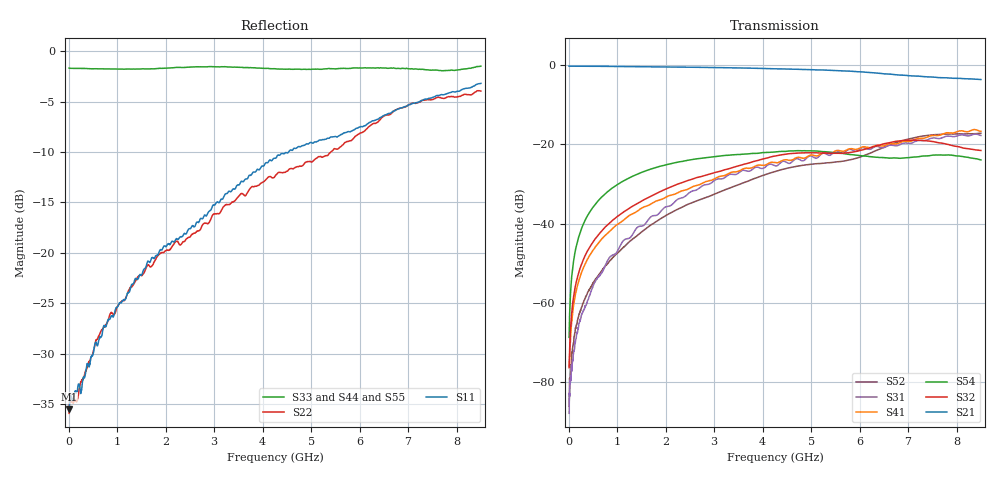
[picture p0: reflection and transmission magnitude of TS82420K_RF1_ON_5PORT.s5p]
!Created with skrf (http://scikit-rf.org).
# GHz S RI R 50.0
!freq ReS11 ImS11 ReS12 ImS12 ReS13 ImS13
! ReS14 ImS14 ReS15 ImS15
! ReS21 ImS21 ReS22 ImS22 ReS23 ImS23
! ReS24 ImS24 ReS25 ImS25
! ReS31 ImS31 ReS32 ImS32 ReS33 ImS33
! ReS34 ImS34 ReS35 ImS35
! ReS41 ImS41 ReS42 ImS42 ReS43 ImS43
! ReS44 ImS44 ReS45 ImS45
! ReS51 ImS51 ReS52 ImS52 ReS53 ImS53
! ReS54 ImS54 ReS55 ImS55
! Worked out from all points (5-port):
!   1601 points, 10 MHz to 8.5 GHz, reference 50 ohm
!   strongest paths, dB at 10 MHz, 2.132 GHz, 4.255 GHz, 6.378 GHz, 8.5 GHz:
!     S21: -0.2, -0.4, -0.9, -2.0, -3.6
!     S32: -76.4, -30.6, -22.9, -20.2, -21.5
!     S54: -68.8, -24.8, -21.9, -23.2, -23.9
!     S41: -76.0, -32.8, -24.5, -20.2, -16.7
!     S31: -88.0, -35.2, -25.4, -20.5, -17.7
!     S52: -86.2, -37.1, -26.9, -21.3, -17.2
!   lowest |S11| = -35.6 dB at 10 MHz (marker M1), VSWR 1.03, Z = 51.7 + j0.0121 ohm
!   |S11| at or under -10 dB: start of sweep to 4.532 GHz
